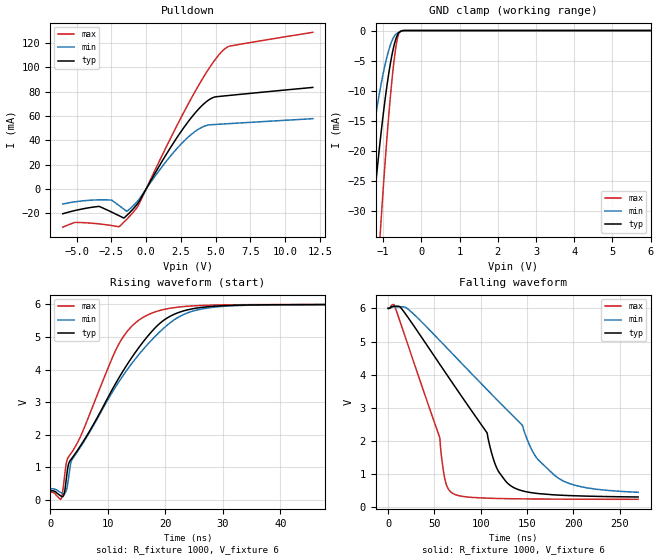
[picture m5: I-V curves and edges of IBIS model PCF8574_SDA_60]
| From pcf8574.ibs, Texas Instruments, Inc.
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[Model]   PCF8574_SDA_60
Model_type  I/O_open_drain
Vinl=1.8
Vinh=4.2
Enable   Active-Low
Vref =   6.0
Rref =   4700
Cref =   10p
Vmeas =   3.0
| variable   typ   min   max
C_comp   2.20pF   1.72pF   2.47pF
| C_pulldown   1.21pF   1.02pF   1.47pF
| C_tri-state   2.20pF   1.72pF   2.47pF
[Temperature Range]   40   100   -40
| Ambient temperature   25   85   -40
[Voltage range]   6   6   6
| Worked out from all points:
|   slope of the pulldown table from 0 to 0.9 V, typ, clamps not added: 50.1 ohm
|   GND clamp passes 1 mA (typ) near -0.65 V on its own axis
|   rising waveform, R_fixture 1000, V_fixture 6: 20-80 % time 11.8ns typ, 12.7ns min, 8.66ns max; typ from 0.281 V to 6 V
|   falling waveform, R_fixture 1000, V_fixture 6: 20-80 % time 71.2ns typ, 98ns min, 36.2ns max; typ from 6 V to 0.31 V
[GND Clamp]
| PCF8574_SDA_60
|   Voltage   I(typ)   I(min)   I(max)
-6V       -559.2mA   -418.5mA   -811.8mA
-1.555V   -51.46mA   -33.82mA   -88.02mA
-1.525V   -49.1mA    -31.75mA   -84.27mA
-1.395V   -39.26mA   -23.03mA   -68.46mA
-1.32V    -33.87mA   -19.46mA   -59.71mA
-1.285V   -31.44mA   -17.9mA    -55.72mA
-1.075V   -18.11mA   -9.582mA   -33.46mA
-890mV    -8.629mA   -4.073mA   -16.85mA
-755mV    -3.564mA   -1.468mA   -7.223mA
-650mV    -1.071mA   -508uA     -2.036mA
-545mV    -161.2uA   -143.7uA   -83.41uA
6V        550.7pA    714.2pA    185pA
[Pulldown]
| PCF8574_SDA_60
|   Voltage   I(typ)   I(min)   I(max)
-6V       -20.39mA   -12.39mA   -31.43mA
-5.13V    -17.76mA   -10.6mA    -27.52mA
-3.39V    -14.33mA   -8.976mA   -28.75mA
-1.96V    -21.94mA   -13.55mA   -31.13mA
-1.61V    -23.95mA   -16.56mA   -27.43mA
-1.155V   -19.09mA   -16.2mA    -22mA
-535mV    -10.82mA   -8.878mA   -12.99mA
1.475V    28.91mA    23.15mA    35.19mA
3.065V    55.93mA    43.04mA    70.62mA
4.495V    73.14mA    52.64mA    98.61mA
5.7V      76.63mA    53.57mA    115.6mA
12V       83.56mA    57.82mA    128.9mA
[Ramp]
| PCF8574_SDA_60
| variable   typ   min   max
dV/dt_r   3.54/1.22E-08   3.49/1.30E-08   3.59/9.07E-09
dV/dt_f   3.45/7.23E-08   3.36/9.90E-08   3.53/3.73E-08
R_load = 1000
[Rising Waveform]
| PCF8574_SDA_60
R_fixture =   1000
C_fixture =   0
L_fixture =   0
V_fixture =   6
V_fixture_min = 6
V_fixture_max = 6
|   Time   V(typ)   V(min)   V(max)
0s        281.1mV    341.5mV    236.8mV
1.9ns     111mV      217.2mV    29.9mV
2.4ns     169.9mV    183.3mV    600.4mV
3ns       935.1mV    454.4mV    1.264V
3.8ns     1.288V     1.246V     1.479V
12.8ns    4V         3.855V     5.038V
18.1ns    5.26V      4.998V     5.765V
22.1ns    5.741V     5.594V     5.917V
38.9ns    5.993V     5.989V     5.997V
269.9ns   6V         6V         6V
[Falling Waveform]
| PCF8574_SDA_60
R_fixture =   1000
C_fixture =   0
L_fixture =   0
V_fixture =   6
V_fixture_min = 6
V_fixture_max = 6
|   Time   V(typ)   V(min)   V(max)
0s        6V         6V         6V
10.3ns    6.066V     6.048V     5.816V
55.8ns    4.314V     5.03V      2.098V
61.4ns    4.082V     4.867V     835.9mV
68.5ns    3.79V      4.66V      441.9mV
106.9ns   2.241V     3.547V     273.6mV
117.4ns   1.176V     3.247V     265.3mV
133.7ns   623.3mV    2.786V     256.8mV
185.1ns   365.1mV    855.5mV    244.5mV
269.9ns   309.5mV    450.8mV    238.7mV
